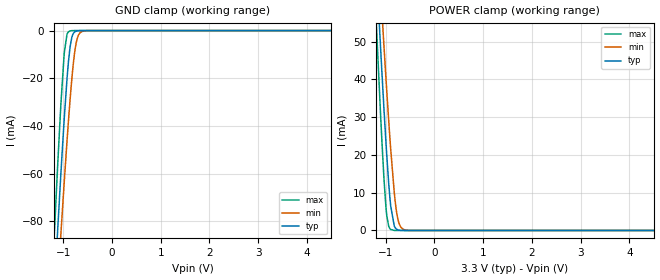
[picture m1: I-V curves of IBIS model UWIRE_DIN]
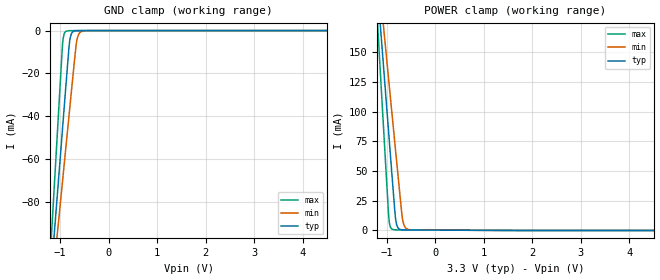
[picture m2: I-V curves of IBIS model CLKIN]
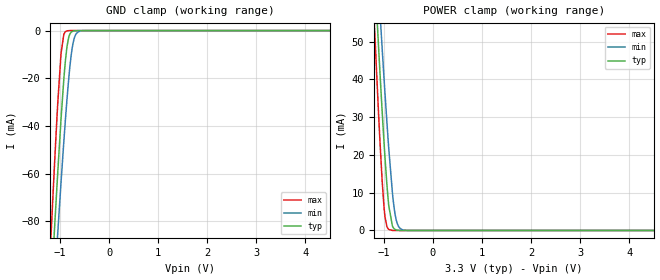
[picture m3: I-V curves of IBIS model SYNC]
| Texas Instruments Incorporated
| Dual Clock Divider Buffer
| Marketing part#   Voltage Range   Package-type   #pins/pkg drawing
| LMK01801   3.15V - 3.45V   LLP   48in SQ
[IBIS Ver]   4.1
[File name]   lmk01801.ibs
[File Rev]   1.1
[Date]   5/08/2012
[Source]   Model built from spectre simulations at:
   Texas Instruments Incorporated.
   Analog-eLab, HPA
   12500 TI Blvd
   Dallas, TX -75243
   For Support e-mail: elab_ibis@list.ti.com
[Notes]   Revision History
   Rev 1.0: 5/08/2012
   -PullUp and Pulldown non-monotonic for LVPECL models
   -Pulldown non-monotonic for LVDS
   -LVPECL simulation recommendation:
   It is recommended that a small (1nF or less) AC coupling cap
   be used. Larger values will result in long settling times
   - C_comp although listed in numberical order of value are obtained from varying PVT conditions.
   For PVT conditions for each specific value, refer to the buffer description under repective [Model].
   IBIS model user is responsible for using appropriate C_comp to simulate for Signal Integrity.
   Rev 1.1: 12/17/2020
   Fixed Syntax issue with Vinh/Vinl in UWIRE_DIN section
[Disclaimer]  This model is designed as an aid for customers of Texas Instruments
 TI and its licensors and suppliers make no warranties, either expressed
 or implied, with respect to this  model, including the warranties of
 merchantability or fitness for a particular purpose.
 The model is provided solely on an "as is" basis. The entire risk as to
 its quality and performance is with the customer.
[Copyright] (C)Copyright 2012 Texas Instruments Incorporated.
   All rights reserved.
[Component]   LMK01801BISQ
[Manufacturer]  Texas Instruments Incorporated
[Package]   |48in LLP SQ package
|   typ   min   max
R_pkg   0   0   0
L_pkg   0   0   0
C_pkg   0   0   0
[Pin]   signal_name   model_name   R_pin   L_pin   C_pin
1   LEUWIRE   UWIRE_DIN
2   CLKOUT0   OSCOUT
3   CLKOUT0*   OSCOUT
4   CLKOUT1*   OSCOUT
5   CLKOUT1   OSCOUT
6   VCC1   POWER
7   CLKOUT2   OSCOUT
8   CLKOUT2*   OSCOUT
9   CLKOUT3*   OSCOUT
10   CLKOUT3   OSCOUT
11   TEST   NC
12   SYNC0   SYNC
13   CLKIN0   CLKIN
14   CLKIN0*   CLKIN
15   VCC2   POWER
16   CLKOUT4   TRI_MODE_OUT
17   CLKOUT4*   TRI_MODE_OUT
18   CLKOUT5*   TRI_MODE_OUT
19   CLKOUT5   TRI_MODE_OUT
20   VCC3   POWER
21   CLKOUT6   TRI_MODE_OUT
22   CLKOUT6*   TRI_MODE_OUT
23   CLKOUT7*   TRI_MODE_OUT
24   CLKOUT7   TRI_MODE_OUT
25   VCC4   POWER
26   Bias   NC
27   EN_PIN_CTRL   SYNC
28   CLKOUT8   TRI_MODE_OUT
29   CLKOUT8*   TRI_MODE_OUT
30   CLKOUT9*   TRI_MODE_OUT
31   CLKOUT9   TRI_MODE_OUT
32   VCC5   POWER
33   CLKOUT10   TRI_MODE_OUT
34   CLKOUT10*   TRI_MODE_OUT
35   CLKOUT11*   TRI_MODE_OUT
36   CLKOUT11   TRI_MODE_OUT
37   VCC6   POWER
38   CLKIN1   CLKIN
39   CLKIN1*   CLKIN
40   SYNC1   SYNC
41   VCC7   POWER
42   CLKOUT12   TRI_MODE_OUT
43   CLKOUT12*   TRI_MODE_OUT
44   CLKOUT13*   TRI_MODE_OUT
45   CLKOUT13   TRI_MODE_OUT
46   VCC8   POWER
47   DATAUWIRE   UWIRE_DIN
48   CLKUWIRE   UWIRE_DIN
[Diff pin]  inv_pin  vdiff  tdelay_typ  tdelay_min  tdelay_max
 2   3   0.0   0.0s   0.0s   0.0s
 4   5   0.0   0.0s   0.0s   0.0s
 7   8   0.0   0.0s   0.0s   0.0s
 9   10   0.0   0.0s   0.0s   0.0s
13   14   0.0   0.0s   0.0s   0.0s
16   17   0.0   0.0s   0.0s   0.0s
18   19   0.0   0.0s   0.0s   0.0s
21   22   0.0   0.0s   0.0s   0.0s
23   24   0.0   0.0s   0.0s   0.0s
28   29   0.0   0.0s   0.0s   0.0s
30   31   0.0   0.0s   0.0s   0.0s
33   34   0.0   0.0s   0.0s   0.0s
35   36   0.0   0.0s   0.0s   0.0s
38   39   0.0   0.0s   0.0s   0.0s
42   43   0.0   0.0s   0.0s   0.0s
44   45   0.0   0.0s   0.0s   0.0s
[Model Selector] TRI_MODE_OUT
LVDS   LVDS OUTPUT
LVPECLLCM   LVPECL 0.7V OUTPUT
LVPECL1P6   LVPECL 1.6V OUTPUT
LVPECL2P0   LVPECL 2.0V OUTPUT
LVCMOS   LVCMOS OUTPUT
[Model Selector] OSCOUT
LVDS   LVDS OUTPUT
LVPECLLCM   LVPECL 0.7V OUTPUT
LVPECL1P6   LVPECL 1.6V OUTPUT
LVPECL2P0   LVPECL 2.0V OUTPUT
[Define Package Model]  llp48_lmk01801_base
[Manufacturer]  Unknown
[OEM]  Unknown
[Description]  Package Model at 5GHz
[Number Of Pins]  49
[Pin Numbers]
1   | DAP:49
2   | L1:1
3   | L2:2
4   | L3:3
5   | L4:4
6   | L5:5
7   | L6:6
8   | L7:7
9   | L8:8
10   | L9:9
11   | L10:10
12   | L11:11
13   | L12:12
14   | L13:13
15   | L14:14
16   | L15:15
17   | L16:16
18   | L17:17
19   | L18:18
20   | L19:19
21   | L20:20
22   | L21:21
23   | L22:22
24   | L23:23
25   | L24:24
26   | L25:25
27   | L26:26
28   | L27:27
29   | L28:28
30   | L29:29
31   | L30:30
32   | L31:31
33   | L32:32
34   | L33:33
35   | L34:34
36   | L35:35
37   | L36:36
38   | L37:37
39   | L38:38
40   | L39:39
41   | L40:40
42   | L41:41
43   | L42:42
44   | L43:43
45   | L44:44
46   | L45:45
47   | L46:46
48   | L47:47
49   | L48:48
[Model Data]
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[End Model Data]
[End Package Model]
| Models and submodels in the file (8): UWIRE_DIN (Input), CLKIN (Input), SYNC (Input), LVDS (Output), LVPECLLCM (Output), LVPECL1P6 (Output), LVPECL2P0 (Output), LVCMOS (Output)
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|   Model   UWIRE_DIN
[Model] UWIRE_DIN
Model_type Input
Vinh = 1.6V
Vinl = 0.4V
C_comp   0.1674p   0.1674pF   0.1674pF
[Voltage Range]   3.3   3.15   3.45
[Temperature Range]   45   125   -40
[Power Clamp Reference]   3.3   3.15   3.45
[GND Clamp Reference]   0   0   0
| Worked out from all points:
|   GND clamp passes 1 mA (typ) near -0.79 V on its own axis
|   POWER clamp passes 1 mA (typ) near -0.82 V on its own axis
[GND Clamp]
|   Voltage   I(typ)   I(min)   I(max)
-3.3V     -965.6mA   -893.6mA   -1.069A
-1.191V   -112.1mA   -132.7mA   -88.59mA
-1.117V   -84.4mA    -107.7mA   -57.4mA
-1.048V   -59.55mA   -84.92mA   -30.5mA
-978.5mV  -36.37mA   -62.95mA   -9.221mA
-924mV    -20.4mA    -46.56mA   -1.598mA
-859.7mV  -6.75mA    -28.81mA   -125.9uA
-795.3mV  -1.278mA   -14.16mA   -6.168uA
-735.9mV  -231.4uA   -5.307mA   -322.1nA
-681.5mV  -39.54uA   -1.674mA   -19.32nA
-577.5mV  -943.2nA   -148.2uA   0A
6.595V    0A         0A         0A
[POWER Clamp]
|   Voltage   I(typ)   I(min)   I(max)
-3.3V     638.8mA    590.5mA    708.3mA
-1.196V   70.39mA    83.75mA    55.37mA
-1.107V   48.47mA    63.9mA     30.8mA
-1.077V   41.42mA    57.43mA    23.19mA
-1.038V   32.31mA    48.95mA    13.93mA
-978.5mV  19.65mA    36.67mA    3.829mA
-899.2mV  6.493mA    21.57mA    264.8uA
-825mV    1.174mA    9.968mA    10.77uA
-765.6mV  254.2uA    3.922mA    572.9nA
-701.3mV  35.15uA    1.11mA     20.98nA
-582.5mV  494.5nA    81.77uA    0A
6.595V    0A         0A         0A
|   Model   CLKIN
[Model]   CLKIN
Model_type   Input
Vinl = 1.7125
Vinh = 1.8875
|   typ   min   max
|   (nom PVT)   (fast PVT)   (slow PVT)
C_comp   0.5966pF   0.57765pF   0.6104pF
[Voltage Range]   3.3   3.15   3.45
[Temperature Range]   45   125   -40
[Power Clamp Reference]   3.3   3.15   3.45
[GND Clamp Reference]   0   0   0
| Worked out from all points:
|   GND clamp passes 1 mA (typ) near -0.75 V on its own axis
|   POWER clamp passes 1 mA (typ) near -0.73 V on its own axis
[GND Clamp]
|   Voltage   I(typ)   I(min)   I(max)
-3.3V     -702.6mA   -596.3mA   -894.5mA
-1.285V   -143.3mA   -147.7mA   -138.8mA
-953.7mV  -47.66mA   -71.87mA   -8.531mA
-933.9mV  -41.92mA   -67.32mA   -3.609mA
-884.4mV  -27.55mA   -55.95mA   -413.2uA
-810.2mV  -6.752mA   -38.87mA   -40.19uA
-775.5mV  -2.224mA   -30.91mA   -27.23uA
-735.9mV  -615.8uA   -21.87mA   -21.67uA
-656.7mV  -62.9uA    -5.145mA   -15.39uA
-612.1mV  -27.35uA   -1.642mA   -12.29uA
-547.8mV  -11.65uA   -311.9uA   -8.099uA
6.595V    0A         0A         0A
[POWER Clamp]
|   Voltage   I(typ)   I(min)   I(max)
-3.3V     1.317A     1.121A     1.677A
-1.256V   236.6mA    250.3mA    219.7mA
-1.068V   137.4mA    171.1mA    85.69mA
-958.7mV  80.14mA    125.2mA    10.37mA
-929mV    64.58mA    112.7mA    3.114mA
-894.3mV  46.51mA    98.19mA    1.056mA
-825mV    11.48mA    69.17mA    515.9uA
-795.3mV  4.573mA    56.79mA    493.7uA
-676.5mV  509.9uA    9.512mA    461.3uA
-632mV    446uA      3.2mA      450.9uA
-567.6mV  418.6uA    890.8uA    436.1uA
6.595V    0A         0A         0A
|   Model   SYNC
[Model]   SYNC
Model_type   Input
Vinl = 0.4
Vinh = 1.2
|   typ   min   max
|   (nom PVT)   (fast PVT)   (slow PVT)
C_comp   0.1841pF   0.1807pF   0.1863pF
[Voltage Range]   3.3   3.15   3.45
[Temperature Range]   45   125   -40
[Power Clamp Reference]   3.3   3.15   3.45
[GND Clamp Reference]   0   0   0
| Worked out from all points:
|   GND clamp passes 1 mA (typ) near -0.79 V on its own axis
|   POWER clamp passes 1 mA (typ) near -0.82 V on its own axis
[GND Clamp]
|   Voltage   I(typ)   I(min)   I(max)
-3.3V     -965.6mA   -893.6mA   -1.069A
-1.191V   -112.1mA   -132.7mA   -88.59mA
-1.117V   -84.4mA    -107.7mA   -57.4mA
-1.048V   -59.55mA   -84.92mA   -30.5mA
-978.5mV  -36.37mA   -62.95mA   -9.221mA
-924mV    -20.4mA    -46.56mA   -1.598mA
-859.7mV  -6.75mA    -28.81mA   -125.9uA
-795.3mV  -1.278mA   -14.16mA   -6.167uA
-735.9mV  -231.4uA   -5.307mA   -320.6nA
-681.5mV  -39.54uA   -1.674mA   -17.85nA
-577.5mV  -941.8nA   -148.2uA   0A
6.595V    0A         0A         0A
[POWER Clamp]
|   Voltage   I(typ)   I(min)   I(max)
-3.3V     638.8mA    590.5mA    708.3mA
-1.196V   70.39mA    83.75mA    55.37mA
-1.107V   48.47mA    63.9mA     30.8mA
-1.077V   41.42mA    57.43mA    23.19mA
-1.038V   32.31mA    48.95mA    13.93mA
-978.5mV  19.65mA    36.67mA    3.829mA
-899.2mV  6.493mA    21.57mA    264.8uA
-825mV    1.174mA    9.968mA    10.77uA
-765.6mV  254.2uA    3.922mA    572nA
-701.3mV  35.15uA    1.11mA     20.08nA
-582.5mV  493.7nA    81.77uA    0A
6.595V    0A         0A         0A
